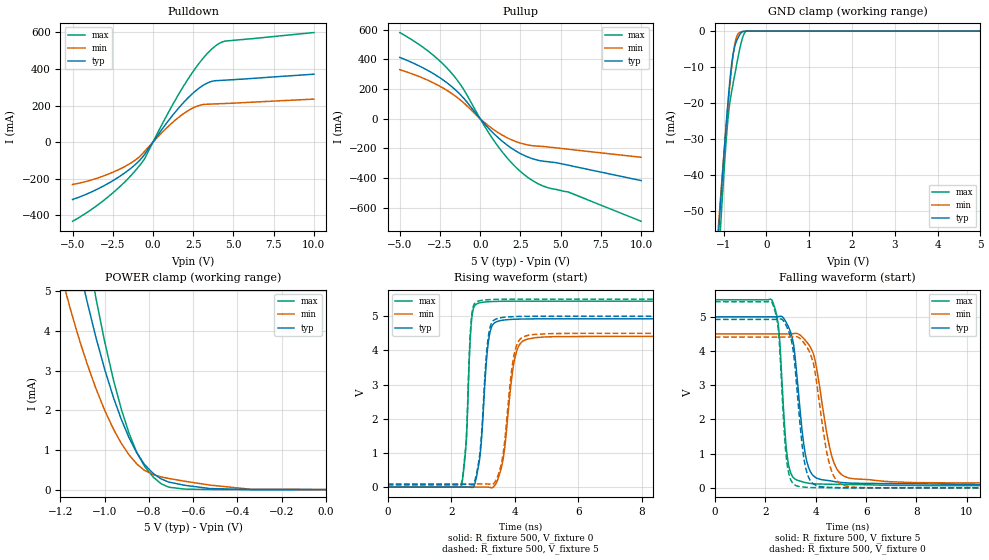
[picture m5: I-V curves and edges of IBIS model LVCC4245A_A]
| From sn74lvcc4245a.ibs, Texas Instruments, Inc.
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[Model]   LVCC4245A_A
Model_type  I/O
Vinl=0.8
Vinh=2.0
Enable   Active-Low
Vref =   0
Rref =   500
Cref =   50p
Vmeas =   2.5
| variable   typ   min   max
C_comp   11.0pF   NA   NA
| C_pullup   9.06pF   6.94pF   10.71pF
| C_pulldown   9.09pF   6.34pF   12.30pF
| C_tri-state   5.59pF   4.88pF   6.81pF
[Temperature Range]   40   100   -40
| Ambient temperature   25   85   -40
[Voltage range]   5   4.5   5.5
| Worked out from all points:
|   slope of the pulldown table from 0 to 0.75 V, typ, clamps not added: 8.1 ohm
|   slope of the pullup table from 0 to 0.75 V, typ, clamps not added: 8.38 ohm
|   GND clamp passes 1 mA (typ) near -0.62 V on its own axis
|   POWER clamp passes 1 mA (typ) near -0.86 V on its own axis
|   rising waveform, R_fixture 500, V_fixture 0: 20-80 % time 218ps typ, 311ps min, 145ps max; typ from 0 V to 4.92 V
|   falling waveform, R_fixture 500, V_fixture 5: 20-80 % time 418ps typ, 616ps min, 276ps max; typ from 5 V to 0.077 V
|   rising waveform, R_fixture 500, V_fixture 5: 20-80 % time 210ps typ, 299ps min, 143ps max; typ from 0.077 V to 5 V
|   falling waveform, R_fixture 500, V_fixture 0: 20-80 % time 385ps typ, 545ps min, 262ps max; typ from 4.92 V to 0 V
[GND Clamp]
| LVCC4245A_A
|   Voltage   I(typ)   I(min)   I(max)
-5V       -860.7mA   -795.6mA   -966.1mA
-1.14V    -60.06mA   -57.45mA   -68.27mA
-1.11V    -54.71mA   -52.59mA   -62.21mA
-1.08V    -49.43mA   -47.8mA    -56.24mA
-1.05V    -44.23mA   -43.08mA   -50.38mA
-915mV    -22.36mA   -23.09mA   -26.78mA
-870mV    -16.02mA   -17.1mA    -21.36mA
-820mV    -10.09mA   -11.1mA    -17.36mA
-720mV    -3.525mA   -2.612mA   -10.93mA
-615mV    -849.1uA   -285.5uA   -4.566mA
-475mV    -8.999uA   -49.26uA   -38.82uA
5V        34.78pA    95.12uA    412.6pA
[POWER Clamp]
| LVCC4245A_A
|   Voltage   I(typ)   I(min)   I(max)
-5V       323.2mA    258.5mA    441.8mA
-1.185V   7.567mA    5.174mA    10.02mA
-1.155V   6.702mA    4.557mA    8.81mA
-1.08V    4.756mA    3.185mA    6.103mA
-1.04V    3.848mA    2.556mA    4.848mA
-1V       3.034mA    2.001mA    3.732mA
-960mV    2.318mA    1.522mA    2.76mA
-890mV    1.31mA     876.2uA    1.424mA
-820mV    632.7uA    485.2uA    588uA
-745mV    271uA      320.5uA    147.7uA
-525mV    26.96uA    114.4uA    1.262uA
-84.45fV  34.78pA    232.5pA    575.7pA
[Pulldown]
| LVCC4245A_A
|   Voltage   I(typ)   I(min)   I(max)
-5V       -313mA     -231.2mA   -432.1mA
-3.855V   -273.3mA   -207.2mA   -369.3mA
-2.74V    -223.1mA   -173.3mA   -295.2mA
-1.72V    -165.6mA   -131.6mA   -214.5mA
-905mV    -106.1mA   -84.61mA   -135.4mA
-500mV    -64.09mA   -48.45mA   -87.29mA
840mV     103.2mA    76.72mA    142.6mA
1.915V    217.5mA    156.4mA    307.4mA
2.98V     302mA      203mA      443.1mA
3.85V     335.2mA    208.8mA    522.7mA
4.535V    338.8mA    211.2mA    552.3mA
10V       371mA      235mA      598.3mA
[Pullup]
| LVCC4245A_A
|   Voltage   I(typ)   I(min)   I(max)
-5V       412.5mA    329.9mA    579.7mA
-3.215V   322.5mA    257.1mA    453mA
-2.48V    273.7mA    217.2mA    385.4mA
-1.835V   221.8mA    174.7mA    313.6mA
-1.045V   140.3mA    108.8mA    199.7mA
215mV     -27.36mA   -20.48mA   -39.65mA
1.03V     -118.7mA   -87.13mA   -174.3mA
1.91V     -195.5mA   -139.7mA   -291.9mA
2.79V     -249.5mA   -172.2mA   -380.8mA
3.915V    -285.4mA   -186.4mA   -452.6mA
5.475V    -312.3mA   -204.9mA   -492.8mA
10V       -415.7mA   -259mA     -689.7mA
[Ramp]
| LVCC4245A_A
| variable   typ   min   max
dV/dt_r   2.96/2.26E-10   2.66/3.21E-10   3.27/1.45E-10
dV/dt_f   2.97/4.26E-10   2.66/6.38E-10   3.27/2.83E-10
R_load = 500
[Rising Waveform]
| LVCC4245A_A
R_fixture =   500
C_fixture =   0
L_fixture =   0
V_fixture =   0
V_fixture_min = 0
V_fixture_max = 0
|   Time   V(typ)   V(min)   V(max)
0s        153.5pV    3.439nV    1.424nV
2.305ns   -66.75uV   10.68uV    -827.2uV
2.475ns   1.03mV     -31.95uV   1.396V
2.65ns    -10.7mV    -66.06uV   4.992V
3.035ns   2.713V     1.155mV    5.414V
3.295ns   4.74V      -15.68mV   5.43V
3.62ns    4.884V     771.2mV    5.438V
4.05ns    4.914V     3.959V     5.441V
4.67ns    4.923V     4.375V     5.442V
50ns      4.924V     4.409V     5.442V
[Falling Waveform]
| LVCC4245A_A
R_fixture =   500
C_fixture =   0
L_fixture =   0
V_fixture =   5
V_fixture_min = 4.5
V_fixture_max = 5.5
|   Time   V(typ)   V(min)   V(max)
0s        5V         4.5V       5.5V
2.265ns   4.999V     4.5V       5.479V
2.53ns    5.007V     4.5V       4.649V
2.79ns    4.886V     4.499V     1.521V
2.925ns   4.693V     4.498V     658.6mV
3.125ns   4.165V     4.51V      287.6mV
3.72ns    590.4mV    4.191V     134.6mV
4.685ns   192.3mV    812.9mV    103.8mV
5.535ns   135.2mV    263.1mV    97.25mV
50ns      76.79mV    91.17mV    61.99mV
[Rising Waveform]
| LVCC4245A_A
R_fixture =   500
C_fixture =   0
L_fixture =   0
V_fixture =   5
V_fixture_min = 4.5
V_fixture_max = 5.5
|   Time   V(typ)   V(min)   V(max)
0s        76.79mV    91.15mV    61.99mV
2.305ns   76.72mV    91.16mV    61.49mV
2.47ns    77.73mV    91.11mV    1.418V
2.645ns   66.15mV    91.08mV    5.045V
3.005ns   2.368V     92.19mV    5.47V
3.275ns   4.816V     70.35mV    5.488V
3.6ns     4.962V     800.2mV    5.496V
4.01ns    4.99V      4.009V     5.499V
4.61ns    4.998V     4.467V     5.5V
50ns      5V         4.5V       5.5V
[Falling Waveform]
| LVCC4245A_A
R_fixture =   500
C_fixture =   0
L_fixture =   0
V_fixture =   0
V_fixture_min = 0
V_fixture_max = 0
|   Time   V(typ)   V(min)   V(max)
0s        4.924V     4.409V     5.442V
2.27ns    4.923V     4.409V     5.411V
2.515ns   4.929V     4.409V     4.611V
2.88ns    4.658V     4.407V     617.4mV
3.115ns   3.97V      4.418V     115.3mV
3.355ns   2.028V     4.38V      37.83mV
3.78ns    221.3mV    3.931V     11.26mV
4.56ns    13.4mV     654.4mV    5.157mV
5.31ns    3.639mV    36.2mV     1.454mV
50ns      287.5nV    2.426uV    123.9nV
